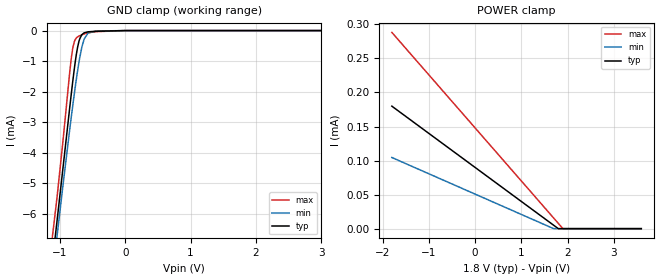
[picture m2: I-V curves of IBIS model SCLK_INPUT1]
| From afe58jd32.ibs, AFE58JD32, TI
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|   Model
[Model]   SCLK_INPUT1
Model_type   Input
Vinl = 0.45
Vinh = 1.35
|   typ   min   max
C_comp   1.431pF   1.417pF   1.444pF
[Voltage Range]   1.8   1.7   1.9
[Temperature Range]   25   85   -40
[Power Clamp Reference]   1.8   1.7   1.9
[GND Clamp Reference]   -0   -0   -0
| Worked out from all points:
|   GND clamp passes 1 mA (typ) near -0.76 V on its own axis
[GND Clamp]
|   Voltage   I(typ)   I(min)   I(max)
-1.8V     -19.89mA   -21.53mA   -17.48mA
-1.201V   -9.15mA    -9.671mA   -8.298mA
-1.044V   -6.224mA   -6.724mA   -5.449mA
-1.039V   -6.122mA   -6.624mA   -5.344mA
-849.6mV  -2.504mA   -3.224mA   -1.342mA
-806.4mV  -1.705mA   -2.495mA   -607.9uA
-768.6mV  -1.066mA   -1.888mA   -305uA
-709.2mV  -350.5uA   -1.034mA   -179.2uA
-633.6mV  -79.25uA   -302.4uA   -113.3uA
-568.8mV  -40.36uA   -78.6uA    -72.34uA
-433.8mV  -22.13uA   -14.27uA   -35.08uA
3.595V    0A         0A         0A
[POWER Clamp]
|   Voltage   I(typ)   I(min)   I(max)
-1.8V     179.9uA    104.5uA    288.3uA
1.699V    5.033uA    18.52nA    15.64uA
1.796V    175.1nA    0A         8.067uA
1.899V    0A         0A         73.64nA
3.595V    0A         0A         0A
